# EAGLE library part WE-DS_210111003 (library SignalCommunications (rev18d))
WE-DS D-SUB-Filter, Solder Pin Straight Characteristics Standard type filtered with 1000 pF High attenuation: max. ≥ 40 dB @ 180 MHz Choice of UNC 4/40 or through hole Rated voltage: 100 VDC Rated current @ 20 ºC: 5 A Withstand voltage: 250 VRMS Insulation resistance: min. 1000 MΩ Operating temperature: –55 ºC to +125 ºC Applications Filtering of interfaces External connection to -printer -sensor -display Details see: http://katalog.we-online.de/en/pbs/Filter_gerade Created on 2015-05-04 2015 (C) Wurth Elektronik
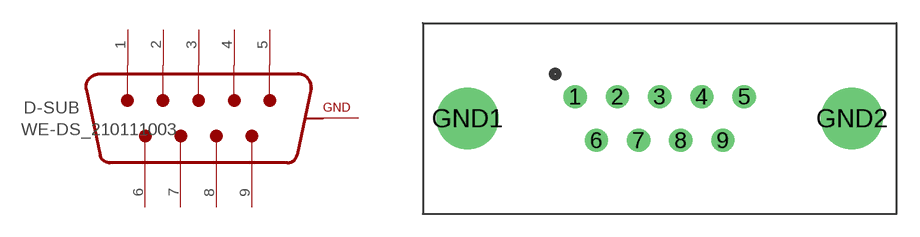
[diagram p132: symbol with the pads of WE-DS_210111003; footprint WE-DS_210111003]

Designator prefix D-SUB

## WE-DS_210111003 (WE-NUMBER: 210111003/9pins_male)  [WE-DS_210111003]
1  1  pas
2  2  pas
3  3  pas
4  4  pas
5  5  pas
6  6  pas
7  7  pas
8  8  pas
9  9  pas
GND1  GND  pwr
GND2  GND  pwr

## Footprint WE-DS_210111003 (pad centres in mm)
drill 1: 1 -5.49,1.42; 2 -2.74,1.42; 3 0,1.42; 4 2.74,1.42; 5 5.49,1.42; 6 -4.11,-1.42; 7 -1.37,-1.42; 8 1.37,-1.42; 9 4.11,-1.42
drill 3: GND1 -12.5,0; GND2 12.5,0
